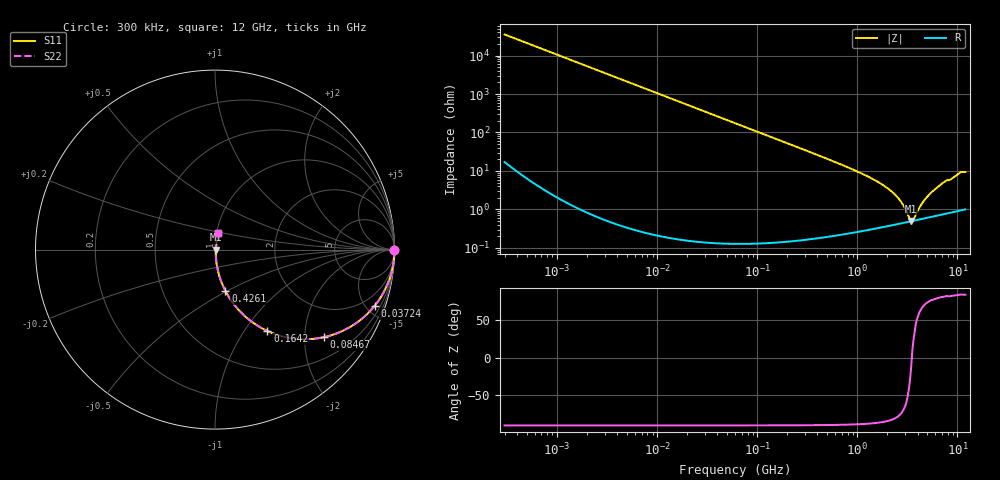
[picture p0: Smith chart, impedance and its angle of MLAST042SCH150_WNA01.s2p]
! MLAST042SCH150_WNA01  S-PARAMETER MODEL  ( General Type )
! Model Generated by TAIYO YUDEN Corporation (http://www.ty-top.com)
! Version 1.0
! TAIYO YUDEN Control No. 150820
! Copyright(c) 2015 TAIYO YUDEN CO.,LTD. All Rights Reserved.
! Product Description (link to TY-COMPAS)
! https://ds.yuden.co.jp/TYCOMPAS/or/detail?pn=MLAST042SCH150JWNA01&u=M
! Products Name : Multilayer Ceramic Capacitors
! Characteristics :
!  Capacitance : 15 pF , Rated Voltage : 25V , TCC : CH / C0H
!  Case Size : 0.4 x 0.2 / 0.016 x 0.008 [mm/inch] , Thickness : 0.2 / 0.008 [mm/inch]
!  (Conditions: Temperature = 25 degC , DC Bias Current/Voltage = 0A / 0V)
! External Node Assignments :
!  1  o---| |---o  2
! GND o---------o GND
! Frequency Range : 0.3MHz  -  12000MHz  [ 401 STEP ]
# MHz S RI R 50
! Freq[MHz].  S11 Real  S11 Imag  S21 Real  S21 Imag  S12 Real  S12 Imag  S22 Real  S22 Imag
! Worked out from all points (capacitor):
!   401 points, 300 kHz to 12 GHz, reference 50 ohm
!   read as one part in series: C = 15.1 pF near 316.3 kHz
!   lowest |Z| = 504 mohm at 3.455 GHz (marker M1)
!   series resonance near 3.501 GHz, so ESL is about 140 pH
!   S11 on the Smith chart (normalised r, x): 300 kHz: open; 37.24 MHz: 1.00, -5.67; 84.67 MHz: 1.00, -2.49; 164.2 MHz: 1.00, -1.28; 426.1 MHz: 1.00, -0.49; 12 GHz: 1.02, +0.19
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0.3  1 -0.00284  9.46e-06 0.00284  9.46e-06 0.00284  1 -0.00284
1.769972  0.9997 -0.0168  0.000284 0.0168  0.000284 0.0168  0.9997 -0.0168
10.44266  0.9903 -0.098  0.00971 0.098  0.00971 0.098  0.9903 -0.098
21.92581  0.9586 -0.1991  0.0414 0.1991  0.0414 0.1991  0.9586 -0.1991
37.24419  0.8891 -0.3137  0.1109 0.3137  0.1109 0.3137  0.8891 -0.3137
60  0.7555 -0.4294  0.2445 0.4294  0.2445 0.4294  0.7555 -0.4294
84.66778  0.6081 -0.4877  0.3919 0.4877  0.3919 0.4877  0.6081 -0.4877
164.1901  0.2919 -0.4536  0.7081 0.4536  0.7081 0.4536  0.2919 -0.4536
353.9943  0.0814 -0.2706  0.9186 0.2706  0.9186 0.2706  0.0814 -0.2706
426.1204  0.0577 -0.2295  0.9423 0.2295  0.9423 0.2295  0.0577 -0.2295
1166.079  0.00918 -0.0796  0.9908 0.0796  0.9908 0.0796  0.00918 -0.0796
2088.533  0.0048 -0.0324  0.9952 0.0324  0.9952 0.0324  0.0048 -0.0324
2650.866  0.00455 -0.017  0.9955 0.017  0.9955 0.017  0.00455 -0.017
2947.191  0.00462 -0.0105  0.9954 0.0105  0.9954 0.0105  0.00462 -0.0105
3276.641  0.0048 -0.00412  0.9952 0.00412  0.9952 0.00412  0.0048 -0.00412
3454.93  0.00492 -0.000952  0.9951 0.000952  0.9951 0.000952  0.00492 -0.000952
3642.919  0.00507 0.00231  0.9949 -0.00231  0.9949 -0.00231  0.00507 0.00231
4623.766  0.00604 0.0156  0.994 -0.0156  0.994 -0.0156  0.00604 0.0156
5715.274  0.0074 0.0295  0.9926 -0.0295  0.9926 -0.0295  0.0074 0.0295
7448.838  0.0102 0.0512  0.9898 -0.0512  0.9898 -0.0512  0.0102 0.0512
10793.46  0.0177 0.0906  0.9823 -0.0906  0.9823 -0.0906  0.0177 0.0906
12000  0.0184 0.0911  0.9816 -0.0911  0.9816 -0.0911  0.0184 0.0911
